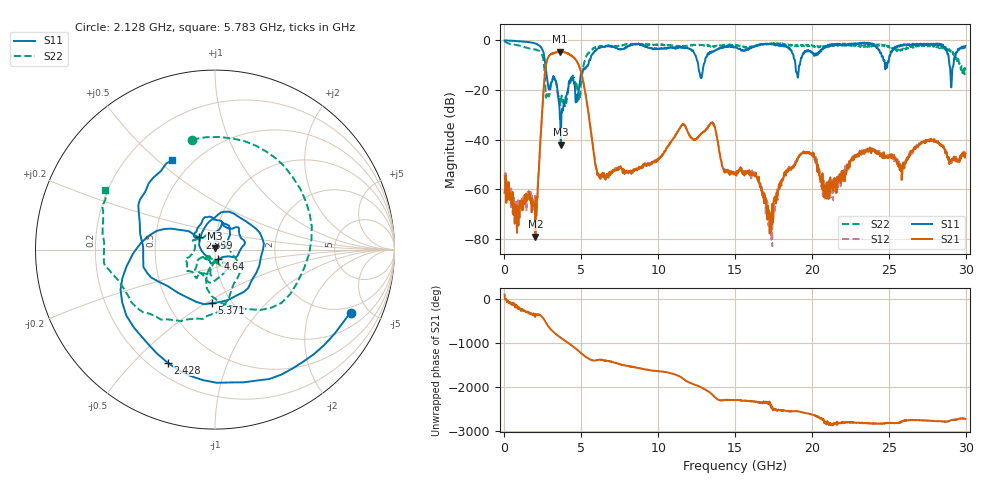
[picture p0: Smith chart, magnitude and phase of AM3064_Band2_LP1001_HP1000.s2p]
# Hz S DB R 50.0
!freq dBS11 angS11 dBS21 angS21 dBS12 angS12 dBS22 angS22
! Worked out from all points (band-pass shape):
!   1600 points, 10 MHz to 29.98 GHz, reference 50 ohm
!   highest |S21| = -4.52 dB at 3.59 GHz (marker M1); lowest = -79.1 dB at 2.016 GHz (marker M2)
!   |S21| within 3 dB of the highest: 2.797 GHz to 4.6 GHz (1.803 GHz wide, 48.8 % of centre)
!   lowest |S11| = -42.1 dB at 3.665 GHz (marker M3), VSWR 1.02, Z = 49.9 + j0.784 ohm
!   |S11| at or under -10 dB: 2.665 GHz to 5.444 GHz (2.778 GHz wide, 68.5 % of centre); 12.61 GHz to 12.96 GHz (349.7 MHz wide, 2.74 % of centre); 28.95 GHz to 29.2 GHz (257.5 MHz wide, 0.886 % of centre)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
!   |S22| runs from -26.5 to -0.3 dB; largest |S21 - S12| = 0.017
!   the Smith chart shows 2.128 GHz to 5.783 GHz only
!   S11 on the Smith chart (normalised r, x): 2.128 GHz: 1.68, -3.83; 2.428 GHz: 0.27, -0.63; 2.859 GHz: 0.83, +0.11; 4.64 GHz: 1.03, -0.11; 5.371 GHz: 0.81, -0.53; 5.783 GHz: 0.39, +0.56
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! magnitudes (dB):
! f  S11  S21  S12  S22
! 10 MHz  -0.1  -61.4  -53.9  -0.3
! 2.016 GHz  -1.3  -79.1  -68.0  -3.7
! 2.128 GHz  -1.6  -63.0  -63.5  -4.1
! 2.428 GHz  -3.3  -31.1  -31.0  -5.9
! 2.859 GHz  -19.1  -6.7  -6.7  -22.5
! 3.59 GHz  -28.7  -4.5  -4.7  -23.7
! 3.665 GHz  -42.1  -4.8  -4.6  -25.0
! 4.64 GHz  -25.0  -7.8  -7.8  -19.0
! 5.015 GHz  -12.9  -13.6  -13.6  -14.9
! 5.371 GHz  -10.5  -25.6  -25.5  -5.9
! 5.783 GHz  -5.2  -44.3  -44.0  -3.1
! 6.27 GHz  -2.7  -54.5  -55.2  -2.6
! 10 GHz  -3.4  -47.7  -47.5  -1.8
! 13.49 GHz  -4.4  -33.2  -33.1  -2.3
! 15 GHz  -2.6  -53.4  -53.9  -1.8
! 16.3 GHz  -2.2  -54.4  -54.8  -2.2
! 17.27 GHz  -1.5  -70.7  -71.3  -1.3
! 19.99 GHz  -4.6  -46.3  -46.1  -1.9
! 20.93 GHz  -2.4  -58.4  -57.4  -2.1
! 25 GHz  -8.3  -47.2  -46.7  -2.3
! 29.08 GHz  -17.7  -48.5  -49.4  -5.2
! 29.98 GHz  -2.2  -45.7  -45.5  -10.9
